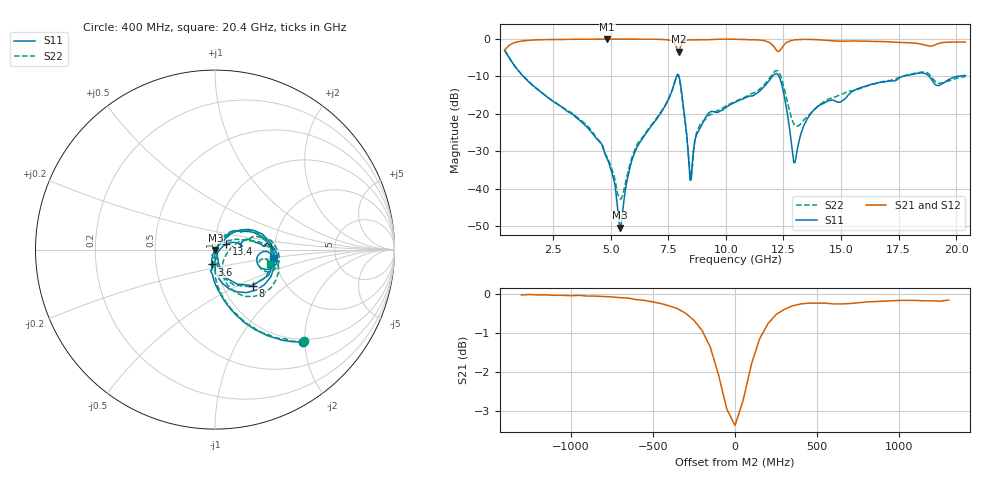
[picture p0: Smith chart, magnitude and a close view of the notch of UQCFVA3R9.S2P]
!  Part Number  UQCFVA3R9  Mounting Orientation: Horizontal
!  Description: Ultra Low ESR Microwave capacitors
!  Application: Coupling, Bypass, Tuning, DC Block
!  Filters, Matching
# GHZ S DB R 50
! Freq  |S11|  S11 Ph  |S21|  S21 Ph  |S12|  S12 Ph  |S22|  S22 Ph
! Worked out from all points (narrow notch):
!   401 points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, 400 MHz to 20.4 GHz, reference 50 ohm
!   highest |S21| = 0.00 dB at 4.85 GHz (marker M1); lowest = -3.4 dB at 7.95 GHz (marker M2)
!   notch at M2: 3.1 dB deep, 218 MHz wide at half that depth
!   lowest |S11| = -50.4 dB at 5.4 GHz (marker M3), VSWR 1.01, Z = 50.2 - j0.223 ohm
!   |S11| at or under -10 dB: 1.214 GHz to 7.863 GHz (6.649 GHz wide, 146 % of centre); 7.968 GHz to 12.02 GHz (4.056 GHz wide, 40.6 % of centre); 12.31 GHz to 17.69 GHz (5.377 GHz wide, 35.8 % of centre)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
!   |S22| runs from -42.8 to -2.9 dB; largest |S21 - S12| = 0.0065
!   S11 on the Smith chart (normalised r, x): 400 MHz: 0.94, -1.97; 3.6 GHz: 0.95, -0.16; 8 GHz: 1.38, -0.60; 13.4 GHz: 1.13, +0.07; 20.4 GHz: 1.93, -0.21
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0.4  -2.94 -46.3  -3.13 43.7  -3.13 43.6  -2.95 -45.8
1.25  -10.23 -78.0  -0.43 12.3  -0.44 12.3  -10.18 -77.0
3.6  -21.44 -103.1  -0.04 -11.1  -0.05 -11.1  -21.18 -94.0
3.75  -22.22 -104.3  -0.03 -12.1  -0.04 -12.1  -21.92 -94.7
4.85  -31.95 -113.4  0.00 -19.1  -0.01 -19.0  -31.59 -89.9
5.4  -50.44 -47.6  -0.01 -22.7  -0.01 -22.7  -42.71 -25.9
6.05  -30.33 48.3  0.00 -27.0  0.00 -27.1  -29.58 54.2
7.1  -20.52 46.0  -0.05 -34.6  -0.05 -34.7  -20.23 50.6
7.95  -9.59 -25.4  -3.36 -35.0  -3.30 -34.9  -9.79 -29.0
8  -10.75 -43.7  -2.71 -27.6  -2.70 -27.8  -10.98 -47.0
8.45  -37.76 -28.5  -0.23 -35.1  -0.21 -35.0  -35.50 -36.5
8.8  -24.75 53.7  -0.19 -38.1  -0.19 -38.2  -23.92 40.2
9.15  -20.70 56.4  -0.17 -40.8  -0.19 -40.8  -21.23 34.6
10.4  -16.93 46.1  -0.06 -49.7  -0.05 -49.6  -16.74 22.8
11.75  -12.13 20.5  -0.57 -62.6  -0.57 -62.6  -11.61 8.4
12.2  -9.21 -25.4  -2.97 -63.5  -2.97 -63.2  -8.42 -27.1
12.5  -14.16 -77.0  -1.73 -47.3  -1.73 -47.4  -12.33 -67.4
12.95  -32.99 -47.2  -0.25 -54.7  -0.24 -54.6  -22.62 -47.8
13.4  -23.00 25.3  -0.07 -60.5  -0.11 -60.5  -21.60 0.2
13.75  -19.48 22.1  -0.12 -63.9  -0.10 -63.9  -19.38 12.8
17.1  -11.21 4.0  -0.74 -84.0  -0.75 -84.1  -11.08 12.0
20.4  -9.75 -8.7  -0.79 -100.2  -0.78 -100.3  -9.97 -15.2
